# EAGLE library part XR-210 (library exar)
FSK MODULATOR/DEMODULATOR
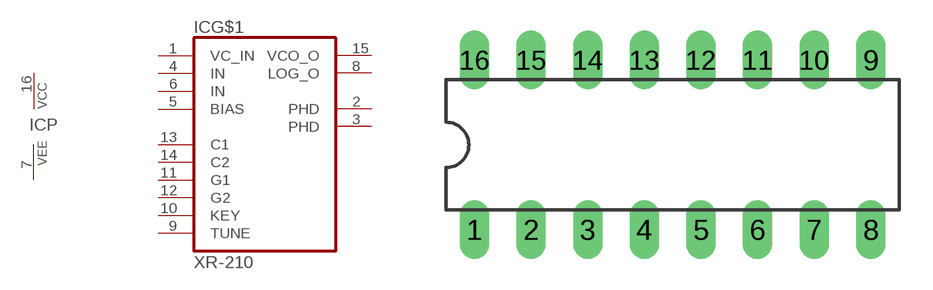
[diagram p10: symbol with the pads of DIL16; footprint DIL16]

Designator prefix IC; gates G$1=XR-210 P=PWR+/-

## XR-210 (OC_FARNELL: unknown; OC_NEWARK: unknown)  [DIL16]
1  G$1:VC_IN  in
2  G$1:PHD  out
3  G$1:PHD  out
4  G$1:IN  in
5  G$1:BIAS  in
6  G$1:IN  in
7  P:VEE  pwr
8  G$1:LOG_O  out
9  G$1:TUNE  in
10  G$1:KEY  in
11  G$1:G1  in
12  G$1:G2  in
13  G$1:C1  in
14  G$1:C2  in
15  G$1:VCO_O  out
16  P:VCC  pwr

## Footprint DIL16 (pad centres in mm)
Dual In Line Package
drill 0.813 long: 1 -8.89,-3.81; 2 -6.35,-3.81; 3 -3.81,-3.81; 4 -1.27,-3.81; 5 1.27,-3.81; 6 3.81,-3.81; 7 6.35,-3.81; 8 8.89,-3.81; 9 8.89,3.81; 10 6.35,3.81; 11 3.81,3.81; 12 1.27,3.81; 13 -1.27,3.81; 14 -3.81,3.81; 15 -6.35,3.81; 16 -8.89,3.81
